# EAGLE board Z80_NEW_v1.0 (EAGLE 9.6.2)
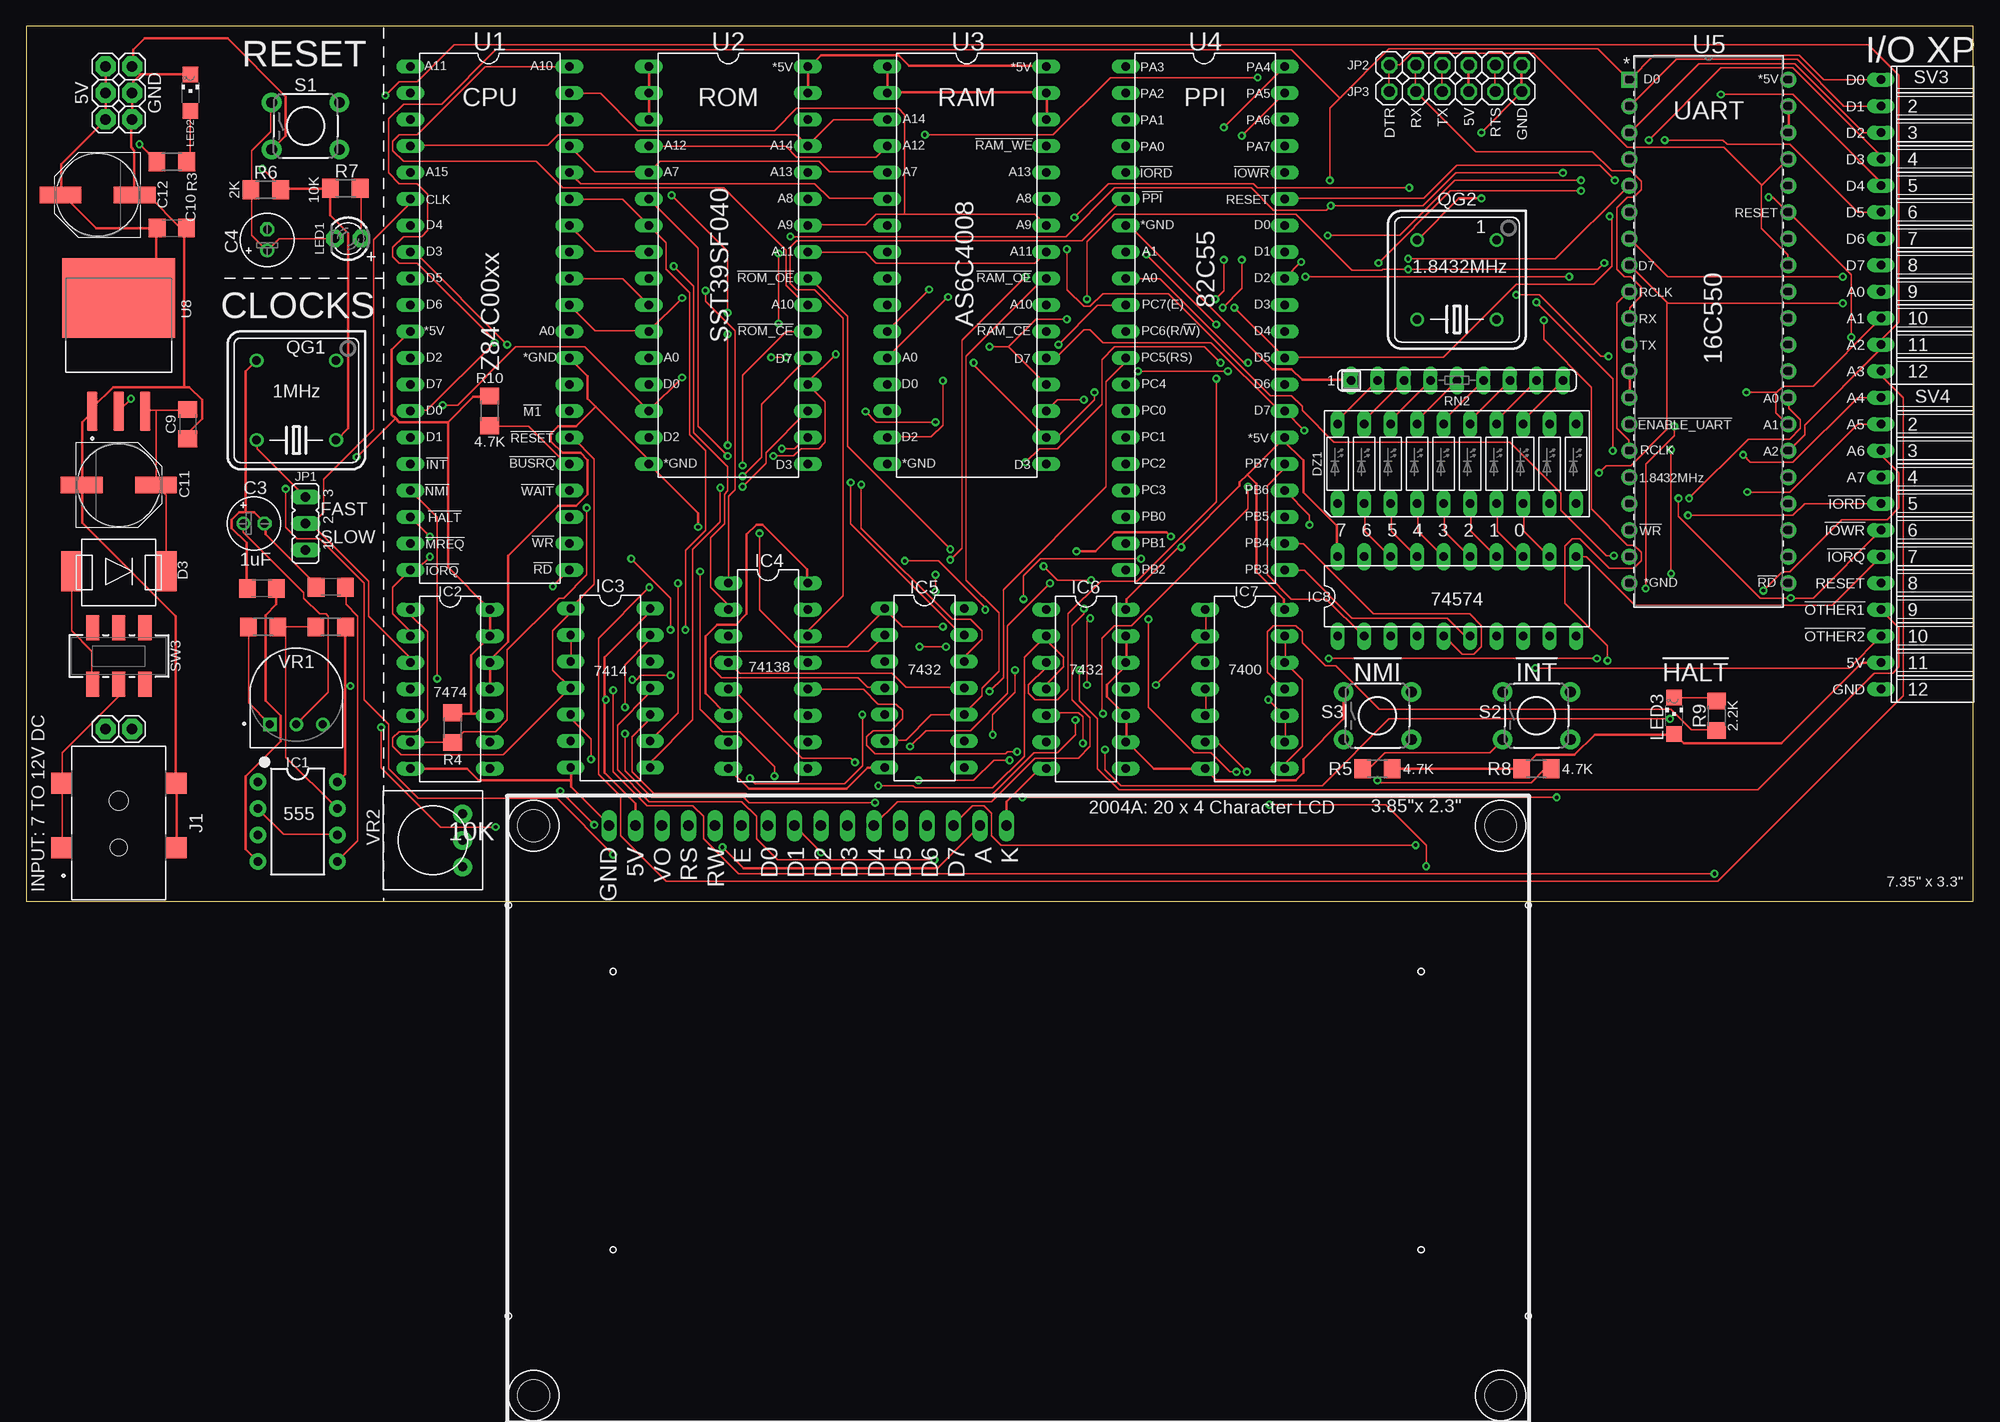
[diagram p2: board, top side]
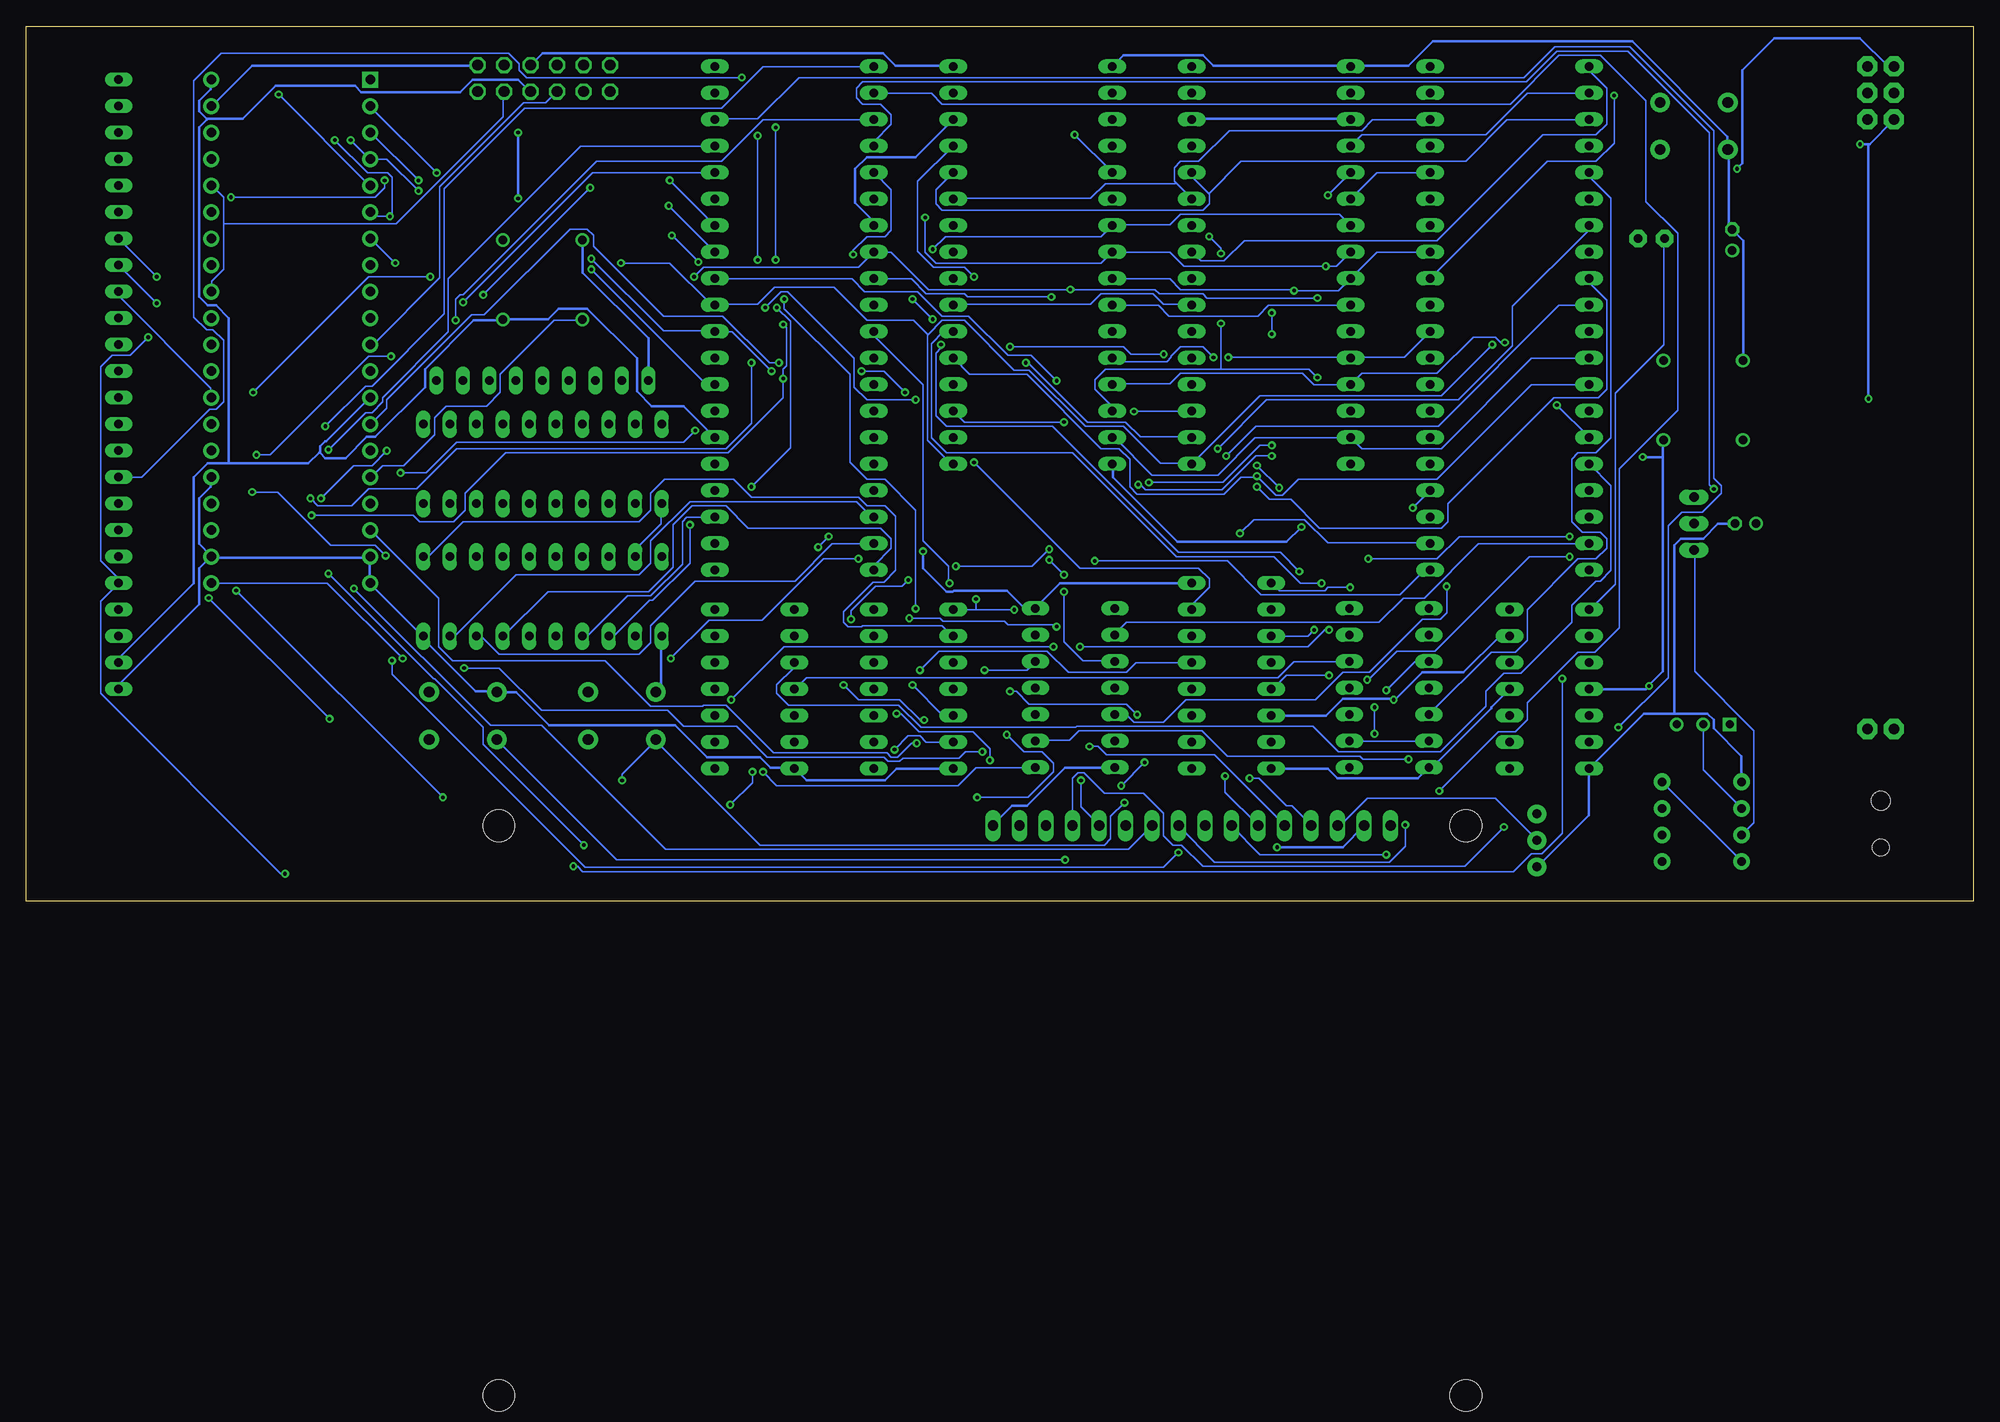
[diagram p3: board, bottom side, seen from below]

Size 186.67 x 83.87 mm. Coordinates in mm from the lower left corner, seen from the top.
Outline: 0,0 186.67,0 186.67,83.87 0,83.87 0,0
Copper layers (1*16): Top 0.035mm / dielectric 0.15mm / Bottom 0.035mm
Design rules "default": minimum track width 6mil, minimum drill 0.35mm, track to track 6mil, track to pad 6mil, pad to pad 6mil, via to via 6mil, smd to smd 6mil, copper to edge 40mil, drill to drill 6mil, minimum pad ring 10mil, minimum via ring 8mil, stop-mask expansion 4mil, vias tented up to drill 0mil, thermal gap 10mil
Net classes: 0 default: clearance 0.254 mm; 3 Power: width 0.254 mm, clearance 0.254 mm
tRestrict: area 17.8,0 to 19,81.3; area 11.4,81.3 to 19.1,82.5; area 0,81.3 to 6.3,82.5
bRestrict: area 17.8,0 to 19,81.3; area 11.4,81.3 to 19.1,82.5; area 0,81.3 to 6.3,82.5

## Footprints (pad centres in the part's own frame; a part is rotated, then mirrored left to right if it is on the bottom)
C1206 = smd 1.6 x 1.8: 1 -1.4,0; 2 1.4,0
E2-5 = drill 0.813 pad 1.27: + -1.016,0 | drill 0.813 pad 1.27 octagon: - 1.016,0
PANASONIC_F = smd 4 x 1.6: + 3.55,0; - -3.55,0
DIODE_5V5A = smd 1.93 x 3.81: A -4.572,0; C 4.572,0
LB10 = drill 0.813 long: 1 -11.43,-3.81; 2 -8.89,-3.81; 3 -6.35,-3.81; 4 -3.81,-3.81; 5 -1.27,-3.81; 6 1.27,-3.81; 7 3.81,-3.81; 8 6.35,-3.81; 9 8.89,-3.81; 10 11.43,-3.81; 11 11.43,3.81; 12 8.89,3.81; 13 6.35,3.81; 14 3.81,3.81; 15 1.27,3.81; 16 -1.27,3.81; 17 -3.81,3.81; 18 -6.35,3.81; 19 -8.89,3.81; 20 -11.43,3.81
DIP08 = drill 0.813 pad 1.626: 1 -3.81,-3.81; 2 -1.27,-3.81; 3 1.27,-3.81; 4 3.81,-3.81; 5 3.81,3.81; 6 1.27,3.81; 7 -1.27,3.81; 8 -3.81,3.81
DIL14 = drill 0.813 long: 1 -7.62,-3.81; 2 -5.08,-3.81; 3 -2.54,-3.81; 4 0,-3.81; 5 2.54,-3.81; 6 5.08,-3.81; 7 7.62,-3.81; 8 7.62,3.81; 9 5.08,3.81; 10 2.54,3.81; 11 0,3.81; 12 -2.54,3.81; 13 -5.08,3.81; 14 -7.62,3.81
DIL16 = drill 0.813 long: 1 -8.89,-3.81; 2 -6.35,-3.81; 3 -3.81,-3.81; 4 -1.27,-3.81; 5 1.27,-3.81; 6 3.81,-3.81; 7 6.35,-3.81; 8 8.89,-3.81; 9 8.89,3.81; 10 6.35,3.81; 11 3.81,3.81; 12 1.27,3.81; 13 -1.27,3.81; 14 -3.81,3.81; 15 -6.35,3.81; 16 -8.89,3.81
DIL20 = drill 0.813 long: 1 -11.43,-3.81; 2 -8.89,-3.81; 3 -6.35,-3.81; 4 -3.81,-3.81; 5 -1.27,-3.81; 6 1.27,-3.81; 7 3.81,-3.81; 8 6.35,-3.81; 9 8.89,-3.81; 10 11.43,-3.81; 11 11.43,3.81; 12 8.89,3.81; 13 6.35,3.81; 14 3.81,3.81; 15 1.27,3.81; 16 -1.27,3.81; 17 -3.81,3.81; 18 -6.35,3.81; 19 -8.89,3.81; 20 -11.43,3.81
SPARKFUN_PRT-12748 = smd 2 x 2: 1_1 -2.35,5.5; 1_2 3.8,5.5; 2 -2.35,-5.5; 3 3.8,-5.5 | hole 1.6: -2.35,0 | hole 1.8: 2.15,0
JP2 = drill 0.914 long: 1 -2.54,0; 2 0,0; 3 2.54,0
1X06 = drill 1.016 octagon: 1 -6.35,0; 2 -3.81,0; 3 -1.27,0; 4 1.27,0; 5 3.81,0; 6 6.35,0
1X01 = drill 1.016 pad 1.93 octagon: 1 0,0
LED3MM = drill 0.813 pad 1.676 octagon: A -1.27,0; K 1.27,0
CHIPLED_1206 = smd 1.5 x 1.5: A 0,-1.75; C 0,1.75
DIL08S = drill 0.813: 1 -3.81,-3.81; 4 3.81,-3.81; 5 3.81,3.81; 8 -3.81,3.81
R1206 = smd 1.6 x 1.803: 1 -1.422,0; 2 1.422,0
SIL9 = drill 0.813 long: 1 -10.16,0; 2 -7.62,0; 3 -5.08,0; 4 -2.54,0; 5 0,0; 6 2.54,0; 7 5.08,0; 8 7.62,0; 9 10.16,0
MOMENTARY_SWITCH = drill 1.016 pad 1.88: 1 -3.251,2.261; 2 3.251,2.261; 3 -3.251,-2.261; 4 3.251,-2.261
FE12W = drill 0.813 long: 1 -13.97,0; 2 -11.43,0; 3 -8.89,0; 4 -6.35,0; 5 -3.81,0; 6 -1.27,0; 7 1.27,0; 8 3.81,0; 9 6.35,0; 10 8.89,0; 11 11.43,0; 12 13.97,0
JS202011SCQN = smd 1.27 x 2.4: 1 -2.5,-2.7; 2 0,-2.7; 3 2.5,-2.7; 4 -2.5,2.7; 5 0,2.7; 6 2.5,2.7
DIL40 = drill 0.813 long: 1 -24.13,-7.62; 2 -21.59,-7.62; 3 -19.05,-7.62; 4 -16.51,-7.62; 5 -13.97,-7.62; 6 -11.43,-7.62; 7 -8.89,-7.62; 8 -6.35,-7.62; 9 -3.81,-7.62; 10 -1.27,-7.62; 11 1.27,-7.62; 12 3.81,-7.62; 13 6.35,-7.62; 14 8.89,-7.62; 15 11.43,-7.62; 16 13.97,-7.62; 17 16.51,-7.62; 18 19.05,-7.62; 19 21.59,-7.62; 20 24.13,-7.62; 21 24.13,7.62; 22 21.59,7.62; 23 19.05,7.62; 24 16.51,7.62; 25 13.97,7.62; 26 11.43,7.62; 27 8.89,7.62; 28 6.35,7.62; 29 3.81,7.62; 30 1.27,7.62; 31 -1.27,7.62; 32 -3.81,7.62; 33 -6.35,7.62; 34 -8.89,7.62; 35 -11.43,7.62; 36 -13.97,7.62; 37 -16.51,7.62; 38 -19.05,7.62; 39 -21.59,7.62; 40 -24.13,7.62
DIL32 = drill 0.813 long: 1 -19.05,-7.62; 2 -16.51,-7.62; 3 -13.97,-7.62; 4 -11.43,-7.62; 5 -8.89,-7.62; 6 -6.35,-7.62; 7 -3.81,-7.62; 8 -1.27,-7.62; 9 1.27,-7.62; 10 3.81,-7.62; 11 6.35,-7.62; 12 8.89,-7.62; 13 11.43,-7.62; 14 13.97,-7.62; 15 16.51,-7.62; 16 19.05,-7.62; 17 19.05,7.62; 18 16.51,7.62; 19 13.97,7.62; 20 11.43,7.62; 21 8.89,7.62; 22 6.35,7.62; 23 3.81,7.62; 24 1.27,7.62; 25 -1.27,7.62; 26 -3.81,7.62; 27 -6.35,7.62; 28 -8.89,7.62; 29 -11.43,7.62; 30 -13.97,7.62; 31 -16.51,7.62; 32 -19.05,7.62
N40A = drill 0.914 pad 1.524 square: 1 -15.24,48.26 | drill 0.914 pad 1.524: 2 -15.24,45.72; 3 -15.24,43.18; 4 -15.24,40.64; 5 -15.24,38.1; 6 -15.24,35.56; 7 -15.24,33.02; 8 -15.24,30.48; 9 -15.24,27.94; 10 -15.24,25.4; 11 -15.24,22.86; 12 -15.24,20.32; 13 -15.24,17.78; 14 -15.24,15.24; 15 -15.24,12.7; 16 -15.24,10.16; 17 -15.24,7.62; 18 -15.24,5.08; 19 -15.24,2.54; 20 -15.24,0; 21 0,0; 22 0,2.54; 23 0,5.08; 24 0,7.62; 25 0,10.16; 26 0,12.7; 27 0,15.24; 28 0,17.78; 29 0,20.32; 30 0,22.86; 31 0,25.4; 32 0,27.94; 33 0,30.48; 34 0,33.02; 35 0,35.56; 36 0,38.1; 37 0,40.64; 38 0,43.18; 39 0,45.72; 40 0,48.26
20X4LCD_2004A = drill 1 long: 1 -41.021,27.94; 2 -38.481,27.94; 3 -35.941,27.94; 4 -33.401,27.94; 5 -30.861,27.94; 6 -28.321,27.94; 7 -25.781,27.94; 8 -23.241,27.94; 9 -20.701,27.94; 10 -18.161,27.94; 11 -15.621,27.94; 12 -13.081,27.94; 13 -10.541,27.94; 14 -8.001,27.94; 15 -5.461,27.94; 16 -2.921,27.94 | hole 3.048: -48.26,-26.67; 44.45,-26.67; 44.45,27.94; -48.26,27.94
TO254P1524X483-4N = smd 3.79 x 0.99: 1 -6.4,2.54; 2 -6.4,0; 3 -6.4,-2.54 | smd 7.62 x 10.84: 4 4.48,0
TRIM_3352T-1-105LF = drill 0.76 pad 1.16 square: 1 -2.54,-2.87 | drill 0.76 pad 1.16: 2 0,-2.87; 3 2.54,-2.87
TRIM-3386 = drill 0.9 pad 1.778: 1 -2.54,-2.857; 2 0,-2.857; 3 2.54,-2.857

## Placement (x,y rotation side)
C1  0.01uF  [C1206]  29.21,30.1 180 top
C2  0.01uF  [C1206]  22.61,29.97 180 top
C3  1uF  [E2-5]  21.84,36.2 0 top
C4  10uF  [E2-5]  23.11,63.37 90 top
C9  100nF  [C1206]  15.49,45.72 270 top
C10  100nF  [C1206]  13.97,64.52 0 top
C11  100uF  [PANASONIC_F]  8.89,39.88 0 top
C12  100uF  [PANASONIC_F]  6.86,67.69 180 top
D3  D1  [DIODE_5V5A]  8.89,31.62 0 top
DZ1  [LB10]  137.16,41.91 0 top
IC1  555  [DIP08]  26.04,7.62 270 top
IC2  74HCT74N  [DIL14]  40.64,20.32 270 top
IC3  74HCT14N  [DIL14]  56.01,20.45 270 top
IC4  74HC138N  [DIL16]  71.12,21.59 270 top
IC5  74S32N  [DIL14]  86.11,20.45 270 top
IC6  7432N  [DIL14]  101.6,20.32 270 top
IC7  74HCT00N  [DIL14]  116.84,20.32 270 top
IC8  74HC574N  [DIL20]  137.16,29.21 0 top
J1  PRT-12748  [SPARKFUN_PRT-12748]  8.89,7.49 90 top
JP1  [JP2]  26.8,36.2 90 top
JP2  [1X06]  137.03,80.14 0 top
JP3  [1X06]  137.03,77.6 0 top
JP17  [1X01]  7.62,77.47 90 top
JP18  [1X01]  10.16,77.47 90 top
JP19  [1X01]  7.62,74.93 90 top
JP20  JP4  [1X01]  7.62,16.51 90 top
JP21  [1X01]  7.62,80.01 90 top
JP22  [1X01]  10.16,80.01 90 top
JP23  [1X01]  10.16,74.93 90 top
JP24  [1X01]  10.16,16.51 90 top
LED1  !RESET!  [LED3MM]  30.86,63.5 180 top
LED2  5v  [CHIPLED_1206]  15.75,77.47 0 top
LED3  !HALT!  [CHIPLED_1206]  157.99,17.78 0 top
QG1  [DIL08S]  25.91,48.01 180 top
QG2  1.8432MHz  [DIL08S]  137.16,59.56 180 top
R1  1k  [R1206]  29.21,26.29 0 top
R2  1k  [R1206]  22.73,26.29 0 top
R3  2K  [R1206]  13.97,70.87 180 top
R4  4.7k  [R1206]  40.89,16.64 90 top
R5  4.7k  [R1206]  129.54,12.7 0 top
R6  10k  [R1206]  22.99,68.2 0 top
R7  2.2k  [R1206]  30.61,68.33 180 top
R8  4.7k  [R1206]  144.78,12.7 0 top
R9  2K  [R1206]  162.05,17.78 270 top
R10  4.7k  [R1206]  44.45,46.99 270 top
RN2  330  [SIL9]  137.16,49.91 0 top
S1  MOMENTARY_SWITCH"  [MOMENTARY_SWITCH]  26.8,74.3 0 top
S2  MOMENTARY_SWITCH"  [MOMENTARY_SWITCH]  144.78,17.78 0 top
S3  MOMENTARY_SWITCH"  [MOMENTARY_SWITCH]  129.54,17.78 0 top
SV3  [FE12W]  177.8,64.77 270 top
SV4  [FE12W]  177.8,34.29 270 top
SW3  JS202011SCQN  [JS202011SCQN]  8.89,23.5 0 top
U1  [DIL40]  44.45,55.88 270 top
U2  SST39SF040_DIP32  [DIL32]  67.31,60.96 270 top
U3  ALLIANCE_AS6C4008  [DIL32]  90.17,60.96 270 top
U4  8255A  [DIL40]  113.03,55.88 270 top
U5  PC16550DN/NOPB  [N40A]  168.91,30.48 0 top
U6  20X4LCD_2004A  [20X4LCD_2004A]  96.9,-20.7 0 top
U8  LM1084ISX-5.0/NOPB  [TO254P1524X483-4N]  8.89,53.34 90 top
VR1  1000k  [TRIM_3352T-1-105LF]  25.91,19.81 0 top
VR2  10k  [TRIM-3386]  38.99,5.84 90 top

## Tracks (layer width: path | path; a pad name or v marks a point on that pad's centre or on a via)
1-100HZ
  Bottom 0.152: JP1.1 26.72,33.63 26.72,22.05 21.03,16.36 21.03,7.52 22.15,6.4 IC1.3
1.8432MHZ
  Bottom 0.152: QG2.5 133.4,55.68 136.04,55.68 141.22,50.49 141.22,48.77 142.54,47.45 146.41,47.45 147.52,46.33 147.52,44.7 150.47,41.76 152.5,41.76 153.62,40.64 U5.16
1MHZ
  Top 0.152: JP1.3 22.15,43.38 22.15,44.2 QG1.5
5V  (via drill 0.35)
  Top 0.254: 55.47,19.3 55.47,12.29 58.42,9.35 U6.2 | 55.47,19.3 55.47,23.37 59.74,27.64 59.74,28.04 IC3.14 | v66.75,5.18 68.78,3.15 87.38,3.15 91.44,7.21 U6.15 | 40.44,45.92 42.88,48.36 44.4,48.36 R10.1 | 40.44,45.92 35.76,45.92 35.41,46.28 | 35.41,46.28 35.05,46.63 35.05,52.83 U1.11 | 42.67,17.98 44.2,17.98 44.4,17.78 IC2.10 | 42.67,17.98 40.95,17.98 R4.2 | 42.67,17.98 42.67,23.57 44.4,25.3 IC2.13 44.5,25.4 44.5,27.94 IC2.14 44.4,28.04 40.44,32 40.44,45.92 | IC4.16 74.88,30.48 74.88,31.8 70.61,36.07 70,36.07 69.09,35.15 69.09,27.53 68.07,26.52 66.24,26.52 65.13,25.4 65.13,19.91 67.26,17.78 IC4.6 | v55.58,19.3 55.47,19.3 | U8.4 8.94,57.91 12.5,61.47 12.5,64.52 C10.1 6.71,64.52 3.45,67.77 C12.+ 3.35,67.77 3.35,70.61 7.62,74.88 JP19.1 JP17.1 JP21.1 | v10.87,72.54 12.5,70.92 R3.2 | v10.06,48.16 8.94,47.04 U8.2 | C2.1 23.98,29.97 23.98,28.45 22.96,27.43 22.96,19.2 24.38,17.78 24.38,15.34 21.03,11.99 21.03,4.98 22.15,3.86 IC1.4 | 30.58,20.62 30.58,12.19 29.87,11.48 IC1.8 | 30.58,20.62 30.58,26.21 R1.2 | 30.58,20.62 v31.09,20.62 | QG1.8 29.77,44.2 30.89,45.31 30.89,64.01 29.16,65.73 29.16,68.17 R7.2 29.16,68.28 24.49,68.28 R6.2 24.49,68.38 v22.66,70.21 | v31.7,42.57 35.41,46.28 | U2.31 74.98,77.52 74.98,79.96 U2.32 75.08,79.96 76.2,81.08 83.62,81.08 84.63,80.06 97.74,80.06 U3.32 | JP3.4 138.28,77.62 138.28,80.06 JP2.4 | R5.2 R8.1 143.46,12.7 144.78,14.02 148.44,14.02 150.37,15.95 157.99,15.95 LED3.A 158.09,15.95 158.9,15.14 168.25,15.14 175.97,22.86 SV4.11 | U5.13 153.72,48.26 153.72,50.8 U5.12 | 110.59,34.09 116.33,39.83 116.33,40.13 117.09,40.89 | 110.59,34.09 105.46,28.96 105.46,27.94 IC6.14
  Top 0.254: 117.09,40.89 U4.26 120.5,44.2 122.43,42.27 122.43,39.22 125.68,35.97 125.68,33.02 IC8.20 | 117.09,40.89 117.96,40.03 117.96,31.6 120.6,28.96 120.6,27.94 IC7.14 | v100.69,33.53 102.51,33.53 104.34,35.36 109.32,35.36 v109.73,34.95 | 110.59,34.09 v110.74,33.93
  Bottom 0.254: v66.75,5.18 60.45,5.18 58.42,7.21 U6.2 | IC4.16 87.58,30.48 89.92,28.14 IC5.14 90.02,28.14 91.03,28.14 92.66,29.77 97.74,29.77 97.84,29.67 98.45,29.67 100.69,31.9 v100.69,33.53 | IC4.6 62.08,17.78 60.45,19.41 55.58,19.41 | 55.58,19.41 55.37,19.41 52.83,21.95 48.87,21.95 45.41,25.4 IC2.13 | v55.58,19.3 55.58,19.41 | 10.06,72.54 9.96,72.54 7.62,74.88 JP19.1 | 10.06,72.54 v10.87,72.54 | 10.06,72.54 v10.06,48.16 | IC2.4 31.39,20.32 v31.09,20.62 31.09,20.73 29.77,22.05 29.77,42.57 | 29.77,42.57 29.77,44.2 QG1.8 | IC1.4 22.25,3.86 29.77,11.38 IC1.8 | v22.66,70.21 22.15,70.71 22.15,79.65 19.1,82.7 10.87,82.7 8.23,80.06 7.62,80.06 JP21.1 | 29.77,42.57 v31.7,42.57 | 169.37,74.98 170.08,75.69 170.08,76.71 168.96,77.83 168.96,78.74 U5.40 | 169.37,74.98 165.91,74.98 162.76,78.13 155.14,78.13 154.53,77.52 145.09,77.52 143.87,78.74 139.5,78.74 138.38,77.62 JP3.4 | JP2.4 137.16,81.28 104.55,81.28 103.33,80.06 97.84,80.06 U3.32 | U4.26 123.65,47.45 126.69,47.45 128.12,48.87 128.12,52.02 132.89,56.79 135.64,56.79 136.65,55.78 140.92,55.78 QG2.8 141.02,55.68 143.76,55.68 148.44,51 148.44,49.28 153.21,44.5 154.03,44.5 156.06,42.47 157.99,42.47 158.5,42.98 | 158.5,42.98 158.5,43.59 157.99,44.09 157.89,44.09 153.72,48.26 U5.13 | SV4.11 177.8,23.27 170.59,30.48 170.59,40.64 169.27,41.96 167.23,41.96 | 167.23,41.96 159.61,41.96 158.6,42.98 158.5,42.98 | 167.23,41.96 167.23,55.88 168.45,57.1 169.27,57.1 170.08,57.91 170.08,74.17 169.37,74.88 169.37,74.98 | v110.74,33.93 v109.73,34.95
12V-0.7V
  Top 0.152: 12.5,47.04 11.48,47.04 U8.3 | 12.5,47.04 15.44,47.04 C9.1 | D3.C 13.41,31.7 13.41,38.91 12.5,39.83 C11.+ 12.5,39.93 12.5,47.04
!BUSRQ!
  Top 0.152: R10.2 44.5,45.52 48.16,45.52 51.71,41.96 52.02,41.96 U1.25
!CTS-RTS!
  Top 0.152: JP3.5 140.82,77.62 140.82,80.06 JP2.5
  Bottom 0.152: 167.74,64.92 167.74,67.46 168.86,68.58 U5.36 | 167.74,64.92 167.74,60.55 168.86,59.44 168.86,58.42 U5.32 | 167.74,64.92 151.18,64.92 140.92,75.18 140.92,77.52 JP3.5
!DSR-DTR!
  Top 0.152: JP3.1 130.66,77.62 130.66,80.06 JP2.1 130.76,80.16 131.67,80.16 132.79,81.28 144.47,81.28 153.52,72.24 162.76,72.24 166.37,68.63 | 166.37,68.63 168.86,71.12 U5.37 | 166.37,68.63 166.32,68.58 166.32,64.52 168.86,61.98 168.86,60.96 U5.33
!ENABLE_IO!
  Top 0.152: IC5.11 89.92,20.52 84.33,20.52 83.01,21.84 68.38,21.84 67.36,22.86 IC4.4
!ENABLE_PPI!
  Top 0.152: IC4.14 74.98,25.4 74.98,25.91 78.33,29.26 78.33,55.88 75.59,58.62 73.86,58.62 73.25,59.23 73.25,62.69 73.86,63.3 101.19,63.3 105.16,67.26 105.36,67.26 U4.6
!ENABLE_UART!  (via drill 0.35)
  Top 0.152: v95.81,42.06 97.13,43.38 98.86,43.38 103.12,47.65 103.12,51.92 104.34,53.14 112.98,53.14 v114.5,51.61
  Bottom 0.152: v95.81,42.06 85.65,31.9 74.27,31.9 73.25,30.89 73.25,30.07 74.88,28.45 74.88,27.94 IC4.15 | v114.5,51.61 115.42,51.61 119.89,56.08 125.58,56.08 132.28,62.79 132.28,63.8 132.89,64.41 134.52,64.41 142.75,56.19 143.97,56.19 152.09,48.06 152.09,47.24 153.62,45.72 U5.14
!HALT!  (via drill 0.35)
  Top 0.152: v38.71,34.95 U1.18 | v58.01,32.82 61.77,29.06 v61.77,26.01 | v88.19,24.38 v85.65,24.38 | v119.08,19.3 120.6,17.78 IC7.10 120.7,17.78 120.7,15.24 IC7.9
  Bottom 0.152: v38.71,34.95 49.28,34.95 51.41,32.82 v58.01,32.82 | v61.77,26.01 62.18,26.01 63.8,24.38 v85.65,24.38 | v88.19,24.38 114,24.38 v119.08,19.3
!INT!
  Bottom 0.152: U1.16 34.75,39.83 34.75,31.7 35.76,30.68 36.17,30.68 38.51,28.35 38.51,26.72 43.38,21.84 45.01,21.84 46.74,20.12 46.74,18.69 51.1,14.33 60.86,14.33 63.3,16.76 85.95,16.76 86.06,16.66 100.89,16.66 103.02,18.8 113.59,18.8 114.71,19.91 114.71,20.73 113.08,22.35 113.08,22.86 IC7.3
!IORD!  (via drill 0.35)
  Top 0.152: v114.1,50.09 114.1,38.3 106.48,30.68 103.02,30.68 99.87,27.53 99.87,20.32 98.86,19.3 96.72,19.3 96.11,19.91 96.11,20.73 97.74,22.35 97.74,22.86 IC6.3 | v107.39,61.98 v114.1,55.27 | SV4.5 170.49,38.1 169.37,36.98 v159.31,36.98
  Bottom 0.152: v114.1,55.27 113.79,54.97 113.79,51.31 114.1,51 v114.1,50.09 114.1,48.26 119.38,42.98 140.72,42.98 144.58,39.12 144.58,37.49 145.69,36.37 148.95,36.37 149.56,36.98 v159.31,36.98 | v107.39,61.98 107.39,62.38 106.07,63.7 104.34,63.7 103.73,64.31 103.73,68.17 U4.5
!IORQ!  (via drill 0.35)
  Top 0.152: IC8.11 149.56,33.02 154.23,28.35 173.13,28.35 SV4.7 | IC2.2 36.78,25.4 36.78,25.91 35.15,27.53 35.15,30.07 U1.20 36.88,31.8 37.49,31.8 v38.71,33.02 | IC4.5 67.77,20.32 74.37,13.72 79.05,13.72 v79.45,13.31 | v81.69,11.07 85.04,11.07 85.24,10.87 92.66,10.87 95.71,13.92 95.71,23.37 97.74,25.4 IC6.2 97.64,25.2 99.47,23.37 99.47,22.45 97.84,20.83 97.84,20.32 IC6.4 | v58.12,21.23 58.52,21.23 58.93,21.64 v61.77,21.64
  Bottom 0.152: v81.69,11.07 v79.45,13.31 | v38.71,33.02 42.57,33.02 51.61,23.98 55.27,23.98 58.01,21.23 v58.12,21.23 | v61.77,21.64 65.84,21.64 67.16,20.32 IC4.5 | IC8.11 148.13,33.02 144.78,36.37 127.91,36.37 126.8,37.49 126.8,39.12 125.48,40.44 118.87,40.44 117.14,38.71 106.88,38.71 106.07,37.9 104.34,37.9 103.33,36.88 103.33,31.7 104.44,30.58 105.46,30.58 108.31,27.74 108.31,26.72 107.9,26.31 106.58,26.31 106.48,26.42 98.86,26.42 97.84,25.4 IC6.2
!IOWR!  (via drill 0.35)
  Top 0.152: v103.43,14.53 103.43,12.6 104.95,11.07 124.26,11.07 130.66,17.48 v157.58,17.48 | SV4.6 171.3,29.06 v169.16,29.06 166.22,29.06 158.39,36.88 v158.39,38.61 | v144.78,57.4 152.09,50.09 v152.09,43.18
  Bottom 0.152: IC6.6 100.38,15.24 100.99,15.85 102.11,15.85 v103.43,14.53 | v169.16,29.06 v157.58,17.48 | v144.78,57.4 132.38,69.8 120.7,69.8 U4.36 | v152.09,43.18 153.52,41.76 155.25,41.76 v158.39,38.61
!MREQ!
  Top 0.152: IC5.4 82.3,20.52 80.67,20.52 79.76,21.44 66.65,21.44 65.63,22.45 65.63,23.27 66.34,23.98 80.77,23.98 82.3,25.5 IC5.2
  Bottom 0.152: U1.19 36.88,34.24 47.45,34.24 52.63,29.06 54.66,29.06 57,26.72 81.18,26.72 82.3,25.6 IC5.2
!NMI!  (via drill 0.35)
  Top 0.152: IC7.6 114.2,15.24 v117.04,12.39 | v119.18,9.25 130.35,9.25 134.21,5.38 v134.21,3.35 | v39.42,21.34 39.42,36.78 U1.17
  Bottom 0.152: v117.04,12.39 117.04,11.38 v119.18,9.25 | v134.21,3.35 133.81,3.35 133.3,2.85 44.09,2.85 42.37,4.57 41.35,4.57 39.42,6.5 v39.42,21.34
!OTHER1!  (via drill 0.35)
  Top 0.152: v100.99,22.15 100.99,19.2 102.72,17.48 102.72,12.7 104.75,10.67 166.01,10.67 177.19,21.84 178.92,21.84 179.53,22.45 179.53,26.21 SV4.9
  Bottom 0.152: IC4.13 80.26,22.86 81.18,21.95 86.77,21.95 88.8,23.98 99.16,23.98 v100.99,22.15
!OTHER2!  (via drill 0.35)
  Top 0.152: IC4.12 80.26,20.32 81.69,18.9 83.41,18.9 84.02,18.29 84.02,17.48 82.91,16.36 81.18,16.36 80.57,15.75 80.57,14.94 81.38,14.12 93.88,14.12 94.08,14.33 v95,14.33 | v144.68,22.35 174.75,22.35 SV4.10
  Bottom 0.152: v95,14.33 96.62,14.33 97.23,13.72 102.62,13.72 102.92,13.41 104.04,13.41 104.44,13.82 115.62,13.82 118.57,16.76 123.65,16.76 125.17,18.29 137.26,18.29 141.33,22.35 v144.68,22.35
!RAM_CE!  (via drill 0.35)
  Top 0.152: v62.48,30.48 62.48,18.09 59.84,15.44 IC3.9
  Bottom 0.152: IC3.6 52.22,15.34 59.74,15.34 IC3.9 | v62.48,30.48 64.52,30.48 67.06,33.02 76.4,33.02 86.36,42.98 98.45,42.98 99.87,44.4 99.87,53.44 98.75,54.56 97.84,54.56 U3.22
!RAM_WE!  (via drill 0.35)
  Top 0.152: v87.17,31.29 v87.17,29.67 | v88.59,32.72 89.71,33.83 89.71,53.75 v95.81,59.84
  Bottom 0.152: v87.17,29.67 87.17,24.89 85.34,23.06 82.3,23.06 IC5.3 | v88.59,32.72 v87.17,31.29 | v95.81,59.84 96.72,60.76 99.67,60.76 101.19,62.28 101.19,68.99 U3.29
!RD!  (via drill 0.35)
  Top 0.152: U1.21 v50.49,30.18 | v91.95,27.94 91.95,28.14 87.48,32.61 v84.23,32.61 | v124.87,23.27 v150.57,23.27 | v106.88,32.82 97.23,32.82 95.61,31.19 v95.61,28.96
  Bottom 0.152: v50.49,30.18 50.49,27.64 51.1,27.03 52.83,27.03 57.91,21.95 60.45,21.95 63.09,19.3 75.49,19.3 77.62,17.17 80.47,17.17 81.18,17.88 82.3,17.88 IC5.5 | v91.95,27.94 95.61,27.94 | 95.61,27.94 IC6.1 | v84.23,32.61 71.53,32.61 68.28,29.36 54.97,29.36 52.63,31.7 52.12,31.7 U1.21 | U5.21 157.78,30.48 v150.57,23.27 | v124.87,23.27 121.21,26.92 116.13,26.92 110.24,32.82 v106.88,32.82 | 95.61,27.94 v95.61,28.96
!RESET!
  Top 0.152: LED1.K 24.28,63.5 23.16,62.38 C4.+ 23.06,62.38 21.64,63.8 21.64,68.17 R6.1 21.64,68.28 21.64,71.93 23.47,73.76 23.47,76.5 S1.1 | IC2.1 36.88,27.94 36.88,27.43 38.51,25.81 38.51,17.37 37.39,16.26 35.76,16.26 35.15,15.65 35.15,14.83 35.97,14.02 45.72,14.02 52.12,20.42 IC3.4 50.49,22.15 50.49,25.91 52.12,27.53 52.12,28.04 IC3.1 52.22,28.14 54.46,30.38 54.46,42.37 52.43,44.4 52.12,44.4 U1.26
  Bottom 0.152: LED1.K 29.67,63.5 29.67,53.34 34.34,48.67 34.34,30.38 36.78,27.94 IC2.1
!ROM-RAM_OE!
  Top 0.152: IC5.6 82.3,15.44 84.33,15.44 86.77,17.88 89.92,17.88 IC5.10 89.92,17.98 91.64,19.71 91.64,20.42 93.27,22.05 93.27,27.64 90.12,30.79 90.12,52.22 97.54,59.64 97.74,59.64 U3.24
!ROM_CE!  (via drill 0.35)
  Top 0.152: v66.55,39.62 66.55,36.37 63.91,33.73 63.91,17.37 59.84,13.31 59.84,12.9 IC3.8 | v68.68,41.76 68.68,50.39 72.85,54.56 74.88,54.56 U2.22
  Bottom 0.152: v68.68,41.76 v66.55,39.62
!ROM_OE!  (via drill 0.35)
  Top 0.152: v116.03,12.39 115.42,12.39 113.59,14.22 111.96,14.22 107.59,18.59 v107.59,27.03 | v102.11,30.79 98.86,30.79 v97.54,32.11 | v88.59,33.73 78.74,43.59 78.74,56.08 75.18,59.64 74.98,59.64 U2.24
  Bottom 0.152: v116.03,12.39 114.71,11.07 97.33,11.07 95.61,12.8 89.92,12.8 IC5.8 | v107.59,27.03 107.59,27.84 105.26,30.18 102.72,30.18 v102.11,30.79 | v97.54,32.11 90.22,32.11 v88.59,33.73
!WAIT!  (via drill 0.35)
  Top 0.152: IC2.6 40.84,15.24 R4.1 40.95,15.24 41.96,16.26 45.01,16.26 46.13,17.37 46.13,24.08 51.1,29.06 51.51,29.06 53.75,31.29 v53.75,37.69
  Bottom 0.152: v53.75,37.69 U1.24
!WR!  (via drill 0.35)
  Top 0.152: v101.7,20.73 101.7,26.82 v102.01,27.13 | v87.88,26.31 84.02,26.31 82.3,28.04 IC5.1 82.3,27.94 78.74,24.38 73.86,24.38 70.31,27.94 v70.31,35.26 | v101.3,15.14 101.3,17.68 100.89,18.09 98.15,18.09 97.84,17.78 IC6.5
  Bottom 0.152: IC6.5 98.75,17.78 v101.7,20.73 | v102.01,27.13 99.06,27.13 98.75,26.82 92.86,26.82 92.56,26.52 88.09,26.52 v87.88,26.31 | v70.31,35.26 68.99,36.58 64.11,36.58 61.87,34.34 52.12,34.34 U1.22 | v101.3,15.14 101.8,15.14 103.12,13.82 103.73,13.82 104.14,14.22 115.01,14.22 119.58,18.8 121.72,18.8 121.82,18.69 126.8,18.69 131.17,23.06 145.8,23.06 147.12,24.38 147.12,29.06 153.62,35.56 U5.18
A0  (via drill 0.35)
  Top 0.152: v88.39,57.91 U3.12 | v72.85,52.12 v71.42,52.12 | v159.41,38.61 165.1,44.3 169.06,44.3 170.08,45.31 170.08,46.13 168.96,47.24 168.96,48.26 U5.28 | v117.14,51.61 116.74,51.61 108.71,59.64 105.46,59.64 U4.9
  Bottom 0.152: SV3.9 177.8,58.01 168.96,49.17 168.96,48.26 U5.28 | U1.30 54.56,52.12 59.64,52.12 U2.12 59.74,52.12 v71.42,52.12 | v88.39,57.91 96.42,57.91 96.72,58.22 100.38,58.22 101.8,59.64 105.36,59.64 U4.9 | v72.85,52.12 73.86,53.14 76,53.14 76.91,52.22 76.91,52.12 77.32,51.71 82.19,51.71 U3.12 | v159.41,38.61 158.7,37.9 155.45,37.9 153.82,39.52 149.25,39.52 145.39,43.38 119.58,43.38 117.14,45.82 v117.14,51.61
A1  (via drill 0.35)
  Top 0.152: SV3.10 171.3,49.38 168.45,49.38 167.79,48.72 | 167.79,48.72 167.74,48.67 167.74,46.84 168.86,45.72 U5.27 | U1.31 54.56,54.66 59.64,54.66 U2.11 v62.89,57.81 | v86.56,58.62 U3.11 | v164.9,48.77 167.74,48.77 167.79,48.72 | v122.63,59.84 v147.93,59.84
  Bottom 0.152: v62.89,57.81 73.46,57.81 73.86,58.22 78.03,58.22 78.44,58.62 v86.56,58.62 100.18,58.62 103.73,62.18 105.36,62.18 U4.8 106.88,60.76 121.72,60.76 v122.63,59.84 | v164.9,48.77 153.82,59.84 v147.93,59.84
A2  (via drill 0.35)
  Top 0.152: U5.26 168.96,43.18 170.49,44.7 170.49,45.62 177.8,52.93 SV3.11 177.8,53.75 179.53,55.47 179.53,79.15 176.58,82.09 41.05,82.09 37.49,78.54 35.76,78.54 v34.44,77.22 | U2.10 57.2,59.64 52.12,59.64 U1.32
  Bottom 0.152: U3.10 82.5,57.1 78.13,57.1 77.11,56.08 68.58,56.08 67.56,57.1 59.74,57.1 U2.10 | v34.44,77.22 34.44,72.64 36.17,70.92 40.84,70.92 U1.32
A3  (via drill 0.35)
  Top 0.152: v65.13,58.52 65.13,57.51 67.97,54.66 67.97,39.42 67.36,38.81 67.36,30.48 IC4.1 | SV3.12 177.8,50.39 179.93,48.26 179.93,19.71 162.15,1.93 61.37,1.93 57,6.3 57,10.06 54.86,12.19 54.86,25.2 v59.74,30.07
  Bottom 0.152: U1.33 52.12,62.18 57.2,62.18 U2.9 60.86,58.52 v65.13,58.52 65.23,58.62 76,58.62 77.01,59.64 82.5,59.64 U3.9 | v59.74,30.07 61.87,30.07 62.18,29.77 66.55,29.77 67.26,30.48 IC4.1
A4  (via drill 0.35)
  Top 0.152: U1.34 54.56,62.28 59.64,62.28 U2.8 | v62.08,60.86 64.01,58.93 64.01,44.91 67.26,41.66 67.26,39.32 66.95,39.01 66.95,36.17 65.63,34.85 65.63,30.07 67.26,28.45 67.26,27.94 IC4.2 | SV4.1 175.56,48.26 169.37,42.06 165.3,42.06 v164.59,42.77 | v151.69,52.22 150.98,52.22 145.09,58.12 v142.85,58.12 | v132.59,68.38 118.06,68.38 117.65,68.78 103.73,68.78 v100.48,65.53
  Bottom 0.152: U2.8 61.06,60.86 v62.08,60.86 75.69,60.86 77.01,62.18 82.5,62.18 U3.8 83.62,61.16 99.47,61.16 100.48,62.18 v100.48,65.53 | v164.59,42.77 163.27,42.77 153.82,52.22 v151.69,52.22 | v132.59,68.38 v142.85,58.12
A5  (via drill 0.35)
  Top 0.152: v63.2,26.01 63.2,33.63 65.13,35.56 65.13,43.18 63.6,44.7 63.6,58.32 61.37,60.55 61.37,63.09 U2.7 57.2,67.26 52.12,67.26 U1.35 | SV4.2 175.56,45.72 169.06,39.22 v165,39.22 | v152.2,33.12 151.49,33.12 147.12,37.49 147.12,39.12 142.24,43.99 125.37,43.99 122.33,47.04 122.33,47.45 121.31,48.46 119.28,48.46 109.53,58.22 103.23,58.22 102.01,57 101.4,57 99.77,58.62 v99.77,62.48
  Bottom 0.152: IC4.3 63.8,25.4 v63.2,26.01 | U2.7 60.76,65.84 76,65.84 77.01,64.82 82.5,64.82 U3.7 83.62,63.7 98.55,63.7 v99.77,62.48 | v165,39.22 162.56,39.22 157.48,34.14 153.21,34.14 v152.2,33.12
A6  (via drill 0.35)
  Top 0.152: IC5.12 89.92,23.37 91.64,25.09 91.64,25.91 90.53,27.03 88.8,27.03 80.06,35.76 v80.06,39.93 | v67.26,42.67 64.41,45.52 64.41,62.59 U2.6 | SV4.3 177.8,42.77 179.53,41.05 179.53,37.69 178.41,36.58 174.04,36.58 169.06,31.6 168.35,31.6 v166.52,29.77 | v95.5,9.96 v146.71,9.96 | v92.66,15.95 92.66,17.88 94.79,20.02 v94.79,22.15 | U1.36 53.14,68.78 75.59,68.78 77.01,67.36 82.5,67.36 U3.6
  Bottom 0.152: v80.06,39.93 79.86,39.93 79.35,39.42 72.03,39.42 68.78,42.67 v67.26,42.67 | v146.71,9.96 v166.52,29.77 | v95.5,9.96 90.63,9.96 88.19,12.39 88.19,13.21 89.31,14.33 91.03,14.33 v92.66,15.95 | v94.79,22.15 90.73,22.15 89.92,22.96 IC5.12 | U2.6 57.2,69.8 52.12,69.8 U1.36
A7  (via drill 0.35)
  Top 0.152: U1.37 54.56,69.9 59.64,69.9 U2.5 60.76,70.92 76,70.92 77.01,69.9 82.5,69.9 U3.5 | v79.05,40.13 79.05,36.17 89.61,25.6 89.92,25.6 IC5.13 | v67.26,54.36 v67.26,43.69 | v67.26,56.39 67.26,62.28 v61.87,67.67 | v118.06,78.94 103.94,78.94 98.45,73.46 v86.16,73.46
  Bottom 0.152: v79.05,40.13 71.93,40.13 68.38,43.69 v67.26,43.69 | v67.26,56.39 v67.26,54.36 | U2.5 v61.87,67.67 | SV4.4 175.56,40.64 169.06,47.14 168.45,47.14 167.74,47.85 167.74,53.75 168.76,54.76 169.37,54.76 170.59,55.98 170.59,78.64 167.94,81.28 140.41,81.28 139.4,80.26 139.4,79.65 138.68,78.94 v118.06,78.94 | U3.5 v86.16,73.46
A8
  Bottom 0.152: U2.27 76.45,68.83 | 76.45,68.83 76.61,68.99 76.61,70.31 76,70.92 74.27,70.92 71.32,73.86 58.62,73.86 57.61,74.88 52.12,74.88 U1.38 | U3.27 97.74,67.36 84.63,67.36 83.21,68.78 76.5,68.78 76.45,68.83
A9
  Top 0.152: 84.23,65.84 96.72,65.84 U3.26 | 84.23,65.84 81.48,65.84 80.47,64.82 74.98,64.82 U2.26 | 84.23,65.84 84.23,75.39 83.62,76 73.86,76 71.73,73.86 58.62,73.86 55.07,77.42 52.12,77.42 U1.39
A10
  Top 0.152: U1.40 52.02,79.96 43.99,79.96 37.49,73.46 35.76,73.46 35.15,72.85 35.15,71.93 36.17,70.92 48.87,70.92 51.41,68.38 66.85,68.38 72.85,62.38 72.85,59.03 74.68,57.2 74.88,57.2 U2.23
  Bottom 0.152: U3.23 97.74,57.2 84.63,57.2 83.62,58.22 78.64,58.22 77.62,57.2 74.98,57.2 U2.23
A11
  Top 0.152: U3.25 96.72,61.16 81.48,61.16 80.47,62.18 74.98,62.18 U2.25
  Bottom 0.152: U2.25 74.07,61.37 71.83,61.37 69.9,63.3 51.41,63.3 41.25,73.46 36.17,73.46 35.15,74.47 35.15,77.93 36.78,79.55 36.78,79.96 U1.1
A12
  Top 0.152: U3.4 81.48,71.32 73.86,71.32 72.85,72.34 59.74,72.34 U2.4
  Bottom 0.152: U2.4 58.62,73.46 46.74,73.46 42.77,77.42 36.88,77.42 U1.2
A13
  Bottom 0.152: 73.3,67.82 73.25,67.77 73.25,66.85 73.86,66.24 98.86,66.24 99.47,66.85 99.47,68.17 U3.28 | 73.3,67.82 74.88,69.39 74.88,69.8 U2.28 | 73.3,67.82 70.21,70.92 48.67,70.92 44.7,74.88 36.88,74.88 U1.3
A14
  Top 0.152: U1.4 36.88,72.44 49.99,72.44 51,73.46 73.86,73.46 U2.29 77.42,74.88 82.5,74.88 U3.3
A15  (via drill 0.35)
  Top 0.152: v54.15,13.61 54.15,15.54 52.22,17.48 52.22,17.88 IC3.5
  Bottom 0.152: v54.15,13.61 58.52,13.61 58.83,13.92 71.53,13.92 73.97,16.36 85.75,16.36 86.67,15.44 89.92,15.44 IC5.9 | IC3.5 46.23,23.88 43.89,23.88 42.77,24.99 42.77,27.94 37.9,32.82 36.17,32.82 35.15,33.83 35.15,34.75 35.76,35.36 37.49,35.36 38.51,36.37 38.51,42.37 37.9,42.98 36.17,42.98 34.75,44.4 34.75,67.36 36.78,69.39 36.78,69.8 U1.5
ADJUST
  Bottom 0.152: U6.3 60.96,7.32 60.66,7.32 58.12,9.86 45.82,9.86 41.86,5.89 VR2.2
CLK
  Top 0.152: IC2.3 36.78,22.86 36.78,23.37 32.82,27.33 32.82,30.68 27.33,36.17 26.82,36.17 JP1.2 27.43,36.17 28.55,37.29 28.55,40.44 33.33,45.21 33.33,63.4 36.78,66.85 36.78,67.26 U1.6
D0  (via drill 0.35)
  Top 0.152: U1.14 36.88,47.04 38.41,47.04 v44.91,53.54 44.81,53.54 44.81,53.85 37.49,61.16 35.76,61.16 35.15,61.77 35.15,62.69 36.17,63.7 37.9,63.7 38.51,64.31 38.51,67.77 37.49,68.78 35.76,68.78 34.75,69.8 34.75,74.98 36.17,76.4 39.83,76.4 45.01,81.58 121.31,81.58 125.93,76.96 | v124.97,69.09 124.97,76 125.93,76.96 | 125.93,76.96 130.66,81.69 150.67,81.69 153.62,78.74 U5.1 153.72,78.74 156.06,81.08 169.98,81.08 172.31,78.74 SV3.1
  Bottom 0.152: v44.91,53.54 45.31,53.54 45.82,54.05 47.95,54.05 51.41,50.6 58.62,50.6 U2.13 59.74,49.48 63.2,49.48 64.31,50.6 76,50.6 77.01,49.58 82.5,49.58 U3.13 | v124.97,69.09 U4.34
D1  (via drill 0.35)
  Top 0.152: v39.93,47.55 41.35,47.55 46.94,53.14 53.54,53.14 U2.14 v62.89,50.19 | v147.32,69.8 137.06,69.8 133.91,66.65 v125.07,66.65 124.66,66.24 119.58,66.24 117.45,68.38 104.34,68.38 99.67,63.7 v73.25,63.7 | SV3.2 174.24,76.2 169.77,80.67 158.19,80.67 153.72,76.2 U5.2 | v72.14,62.08 v72.14,55.37
  Bottom 0.152: v39.93,47.55 U1.15 | 72.14,51 63.7,51 v62.89,50.19 | 72.14,51 83.21,51 84.23,49.99 84.23,49.07 82.6,47.45 82.6,47.04 U3.14 | v125.07,66.65 U4.33 | v147.32,69.8 153.72,76.2 U5.2 | v72.14,55.37 72.14,51 | v72.14,62.08 72.14,62.59 v73.25,63.7
D2  (via drill 0.35)
  Top 0.152: SV3.3 176.17,73.66 169.57,80.26 160.32,80.26 153.72,73.66 U5.3 | v87.88,49.89 87.88,45.62 86.77,44.5 82.6,44.5 U3.15 | v149.05,69.09 136.96,69.09 131.67,63.8 v124.77,63.8 | U4.32 v122.22,61.27
  Bottom 0.152: U3.15 82.5,44.4 82.3,44.4 78.74,40.84 72.44,40.84 68.89,44.4 59.74,44.4 U2.15 58.62,43.38 51,43.38 42.37,52.02 36.88,52.02 U1.12 | v87.88,49.89 90.32,52.32 92.56,52.32 96.32,56.08 98.86,56.08 101.19,58.42 106.27,58.42 107.49,59.64 120.6,59.64 U4.32 | v149.05,69.09 153.62,73.66 U5.3 | v122.22,61.27 v124.77,63.8
D3  (via drill 0.35)
  Top 0.152: SV3.4 177.8,71.42 169.37,79.86 162.46,79.86 v155.55,72.95 | v46.13,53.34 37.29,62.18 36.88,62.18 U1.8 | v149.05,68.07 136.55,68.07 v129.64,61.16
  Bottom 0.152: v155.55,72.95 153.72,71.12 U5.4 152.09,71.12 v149.05,68.07 | 100.23,54.3 100.28,54.25 100.28,44.2 98.04,41.96 97.84,41.96 U3.17 | 100.23,54.3 98.86,55.68 96.72,55.68 91.95,50.9 90.53,50.9 85.14,45.52 81.48,45.52 77.93,41.96 74.98,41.96 U2.17 68.38,48.46 51,48.46 v46.13,53.34 | 100.23,54.3 101.6,55.68 106.07,55.68 109.22,58.83 114.91,58.83 116.53,57.2 120.6,57.2 U4.31 120.7,57.2 121.01,57.2 124.97,61.16 v129.64,61.16
D4  (via drill 0.35)
  Top 0.152: v132.49,61.57 146.61,61.57 153.62,68.58 U5.5 | SV3.5 177.8,68.89 169.37,77.32 v162.46,77.32 | v90.83,51.61 90.83,51.41 U3.18 97.84,44.5 98.86,44.5 102.41,48.06 v102.41,48.77 | v72.44,43.38 73.66,43.38 74.68,44.4 74.88,44.4 U2.18 | v106.58,50.8 v115.21,50.8
  Bottom 0.152: v132.49,61.57 125.58,54.66 120.7,54.66 U4.30 120.6,54.56 118.97,54.56 v115.21,50.8 | v162.46,77.32 153.72,68.58 U5.5 | v90.83,51.61 90.63,51.61 84.94,45.92 81.28,45.92 79.86,44.5 74.98,44.5 U2.18 | v72.44,43.38 67.77,48.06 49.38,48.06 44.2,53.24 44.2,57 36.88,64.31 36.88,64.72 U1.7 | v106.58,50.8 104.44,50.8 v102.41,48.77
D5  (via drill 0.35)
  Top 0.152: v151.79,65.63 151.99,65.43 151.99,60.86 150.27,59.13 142.85,59.13 135.84,52.12 120.7,52.12 U4.29 v115.82,56.9 | SV3.6 175.56,66.04 169.06,72.54 163.07,72.54 162.66,72.95 v157.07,72.95 | v80.47,46.94 81.48,45.92 v87.17,45.92 | v68.68,39.73 70.92,41.96 70.92,42.98 U2.19 | v101.4,48.06 98.86,48.06 U3.19
  Bottom 0.152: U5.6 153.62,66.04 153.21,65.63 v151.79,65.63 151.59,65.84 151.59,69.39 151.99,69.8 153.92,69.8 v157.07,72.95 | v80.47,46.94 74.98,46.94 U2.19 | v87.17,45.92 96.72,45.92 U3.19 | v68.68,39.73 67.46,38.51 65.43,38.51 62.69,35.76 51,35.76 50.39,36.37 50.39,38.1 40.23,48.26 35.97,48.26 35.15,49.07 35.15,57.61 36.78,59.23 36.78,59.64 U1.9 | v115.82,56.9 114.3,58.42 113.69,58.42 107.29,52.02 107.29,49.28 106.07,48.06 v101.4,48.06
D6  (via drill 0.35)
  Top 0.152: v151.28,61.16 150.67,60.55 v132.49,60.55 130.05,60.55 129.95,60.45 127.1,60.45 121.72,65.84 104.34,65.84 101.7,63.2 v101.7,57.71 | v174.14,59.84 157.38,59.84 153.72,63.5 U5.7 | v77.62,52.43 74.98,49.78 74.98,49.58 U2.20 76.61,47.85 76.61,43.99 76,43.38 74.27,43.38 73.56,42.67 v71.63,42.67 | 94.18,53.14 v92.35,53.14 | U3.20 94.18,53.14 | v99.77,55.78 96.83,55.78 94.18,53.14
  Bottom 0.152: v132.49,60.55 121.51,49.58 120.7,49.58 U4.28 | v151.28,61.16 153.62,63.5 U5.7 | v174.14,59.84 SV3.7 | v77.62,52.43 80.77,52.43 81.48,53.14 v92.35,53.14 | v71.63,42.67 68.78,45.52 51.31,45.52 39.73,57.1 36.88,57.1 U1.10 | v99.77,55.78 v101.7,57.71
D7  (via drill 0.35)
  Top 0.152: v68.68,40.74 70.51,42.57 70.51,47.65 U2.21 | v174.14,57.3 157.38,57.3 157.33,57.35 | 157.33,57.35 153.72,60.96 U5.8 | U3.21 97.84,52.12 98.75,52.12 101.4,54.76 102.01,54.76 103.23,53.54 113.59,53.54 120.09,47.04 120.6,47.04 U4.27 v122.53,45.11 | v150.77,41.05 151.49,41.76 153.82,41.76 157.28,45.21 157.28,57.3 157.33,57.35
  Bottom 0.152: U1.13 36.88,49.48 42.37,49.48 51.41,40.44 64.72,40.44 66.24,38.91 66.85,38.91 v68.68,40.74 68.68,40.64 70.21,40.64 71.83,39.01 80.16,39.01 80.87,39.73 80.87,42.37 81.89,43.38 83.62,43.38 90.73,50.49 96.22,50.49 U3.21 | v174.14,57.3 SV3.8 | v150.77,41.05 148.34,41.05 145.39,43.99 123.65,43.99 v122.53,45.11
GND  (via drill 0.35)
  Top 0.254: JP2.6 143.36,80.06 143.36,77.62 JP3.6 143.36,77.52 v139.5,73.66 | U5.38 168.96,73.66 168.96,76.2 U5.39 | U2.3 59.74,74.98 59.74,77.42 U2.2 59.74,77.52 59.74,79.96 U2.1 | U3.1 82.6,79.96 82.6,77.52 U3.2 82.7,77.52 97.74,77.52 U3.31 97.84,77.42 97.84,74.98 U3.30 | RN2.1 127,49.99 122.33,49.99 121.31,51 119.48,51 105.77,64.72 105.46,64.72 U4.7 | v139.5,67.36 137.36,67.36 133.4,63.4 QG2.4 | IC6.7 97.13,12.7 93.98,9.55 U6.16 | IC6.13 105.46,25.4 105.46,22.86 IC6.12 105.36,22.76 105.36,22.45 103.63,20.73 103.63,19.61 105.36,17.88 IC6.10 105.46,17.78 105.46,15.24 IC6.9 105.56,15.24 108.1,12.7 IC7.7 113.08,12.6 114.1,11.58 121.72,11.58 122.43,12.29 122.43,13.61 126.29,17.48 S3.1 | 10.87,79.25 15.75,79.25 LED2.C | 10.87,79.25 10.16,79.96 JP22.1 10.26,80.06 10.26,81.58 11.38,82.7 19.3,82.7 24.89,77.11 24.89,73.36 23.57,72.03 S1.3 | 10.87,79.25 10.87,79.15 10.26,78.54 10.26,77.52 JP18.1 JP23.1 10.06,74.88 10.06,72.24 10.36,71.93 10.36,67.77 C12.- 10.46,67.67 11.68,67.67 14.83,64.52 C10.2 15.14,64.41 15.14,49.28 | J1.2 14.43,5.18 14.43,11.28 J1.3 14.33,11.38 14.33,27.33 5.38,36.27 5.38,39.83 C11.- 5.38,39.93 5.38,45.92 6.3,46.84 U8.1 6.4,47.04 6.4,47.35 8.33,49.28 15.14,49.28 | 15.14,49.28 15.65,49.28 16.87,48.06 16.87,46.23 15.54,44.91 15.54,44.4 C9.2 | 21.03,37.29 21.84,37.29 22.86,36.27 C3.- 22.96,36.17 22.96,35.15 27.74,30.38 27.74,30.18 C1.2 | 21.03,37.29 20.42,37.29 19.71,36.58 19.71,35.76 21.13,34.34 21.13,29.97 C2.2 | 21.03,37.29 21.03,50.8 22.05,51.82 QG1.4 | 54.61,47.4 53.85,48.16 53.85,50.29 U1.29 | 54.61,47.4 59.64,42.37 59.64,41.96 U2.16 64.41,37.19 v64.41,35.87
  Top 0.254: IC2.11 44.5,20.32 44.5,22.86 IC2.12 44.5,22.96 44.5,23.16 46.23,24.89 46.23,33.12 51,37.9 52.73,37.9 53.85,39.01 53.85,42.27 53.14,42.98 51.41,42.98 50.29,44.09 50.29,44.81 51,45.52 52.73,45.52 54.61,47.4 | 52.22,11.58 52.22,10.97 55.88,7.32 U6.1 | 52.22,11.58 52.22,12.8 IC3.7 | IC2.7 42.27,12.7 43.38,11.58 52.22,11.58 | IC5.7 82.3,12.8 80.67,12.8 78.64,10.77 69.29,10.77 67.36,12.7 IC4.8
  Bottom 0.254: JP2.6 143.46,80.06 165,80.06 168.86,76.2 U5.39 | U2.30 74.88,74.98 59.74,74.98 U2.3 | RN2.1 127,53.95 133.3,60.25 133.3,63.3 QG2.4 | U3.30 101.4,71.32 106.07,71.32 107.19,70.21 107.19,66.95 105.46,65.23 105.46,64.82 U4.7 | U3.1 81.48,81.08 73.86,81.08 72.85,80.06 59.74,80.06 U2.1 59.64,80.06 54.15,80.06 51.82,82.4 32.72,82.4 23.57,73.25 23.57,72.14 S1.3 23.47,72.03 23.47,64.72 23.16,64.41 C4.- 23.06,64.31 22.05,63.3 22.05,51.82 QG1.4 | v139.5,67.36 v139.5,73.66 | SV4.12 177.8,20.73 170.08,28.45 170.08,31.9 168.96,33.02 U5.22 | U5.25 168.96,40.64 168.96,39.73 170.08,38.61 170.08,34.24 168.96,33.12 U5.22 | U5.22 168.86,32.92 153.82,32.92 U5.19 153.72,33.02 153.72,30.58 U5.20 153.72,30.48 148.64,25.4 IC8.10 148.54,25.3 148.54,25.09 143.56,20.12 141.53,20.12 S2.1 141.43,20.02 139.7,20.02 136.55,16.87 124.46,16.87 121.41,13.82 116.33,13.82 115.32,12.8 113.08,12.8 IC7.7 112.98,12.7 111.86,11.58 104.34,11.58 103.23,12.7 IC6.7 | IC5.7 82.3,12.8 87.07,12.8 90.73,9.14 92.15,9.14 93.98,7.32 U6.16 | IC8.1 125.78,25.4 125.78,20.62 126.29,20.12 S3.1 | v64.41,35.87 65.84,34.44 76.3,34.44 82.5,40.64 82.5,41.86 U3.16 | VR2.1 41.76,3.35 36.88,8.23 36.88,12.7 IC2.7 36.78,12.8 31.6,17.98 28.65,17.98 | 28.65,17.98 25.5,17.98 24.89,17.37 24.89,16.56 22.25,13.92 22.25,11.48 IC1.1 | IC4.8 61.87,12.7 60.96,11.79 53.24,11.79 IC3.7 52.12,12.9 51.82,12.9 46.23,18.49 46.23,18.59 44.5,20.32 IC2.11 | 28.65,17.98 28.65,34.14 28.04,34.75 25.91,34.75 24.49,36.17 22.86,36.17 C3.-
LED0
  Top 0.152: DZ1.8 143.56,38.1 143.56,35.46 146,33.02 IC8.12
LED1
  Top 0.152: DZ1.7 141.02,38.1 141.02,35.46 143.46,33.02 IC8.13
LED2
  Top 0.152: DZ1.6 138.48,38.1 138.48,35.46 140.92,33.02 IC8.14
LED3
  Top 0.152: DZ1.5 135.94,38.1 135.94,35.46 138.38,33.02 IC8.15
LED4
  Top 0.152: DZ1.4 133.4,38.1 133.4,35.46 135.84,33.02 IC8.16
LED5
  Top 0.152: DZ1.3 130.86,38.1 130.86,35.46 133.3,33.02 IC8.17
LED6
  Top 0.152: DZ1.2 128.32,38.1 128.32,35.46 130.76,33.02 IC8.18
LED7
  Bottom 0.152: DZ1.1 125.78,38.1 125.78,36.17 128.22,33.73 128.22,33.02 IC8.19
N$1
  Top 0.152: R7.1 32.11,68.28 32.11,63.5 LED1.A
N$2
  Top 0.152: 24.89,26.31 27.74,26.31 R1.1 | 24.89,26.31 24.18,26.31 R2.2 24.89,26.31 | 24.89,26.31 24.89,13.82 29.77,8.94 IC1.7
N$3
  Top 0.152: C3.+ 20.83,35.36 26.62,29.57 26.62,29.06 28.14,27.53 28.75,27.53 28.96,27.33 28.96,20.02 25.91,16.97 VR1.2 | IC1.6 29.77,6.4 24.69,6.4 22.25,8.84 IC1.2
  Bottom 0.152: VR1.2 25.91,12.6 22.25,8.94 IC1.2
N$4
  Top 0.152: C1.1 30.68,30.07 30.68,28.45 31.8,27.33 31.8,5.79 29.87,3.86 IC1.5
N$5
  Top 0.152: SW3.1 6.3,20.83 6.3,23.98 4.37,25.91 4.37,31.6 D3.A
N$6
  Top 0.152: R2.1 21.34,26.21 21.34,19 23.37,16.97 VR1.1
N$8
  Top 0.152: J1.1_1 3.45,5.18 3.45,11.28 J1.1_2 3.45,11.38 3.45,14.22 8.84,19.61 8.84,20.73 SW3.2
N$9
  Top 0.152: LED2.A 15.75,71.22 15.44,70.92 R3.1
N$10  (via drill 0.35)
  Top 0.152: v100.58,17.37 100.58,15.95 98.86,14.22 96.62,14.22 92.66,10.26 69.09,10.26 68.99,10.36 60.15,10.36 58.12,12.39 58.12,15.75 59.74,17.37 59.74,17.88 IC3.10 | v108.31,20.73 112.98,25.4 IC7.2 113.08,25.4 113.08,27.94 IC7.1
  Bottom 0.152: v100.58,17.37 100.99,17.37 102.92,19.3 106.88,19.3 v108.31,20.73
N$11
  Top 0.152: DZ1.20 125.78,45.72 125.78,46.13 129.54,49.89 RN2.2
N$12
  Top 0.152: IC7.5 113.08,17.78 113.08,20.32 IC7.4
  Bottom 0.152: IC3.12 59.84,22.96 65.13,22.96 66.65,21.44 111.86,21.44 112.98,20.32 IC7.4
N$13
  Top 0.152: DZ1.19 128.32,45.72 128.32,46.13 132.08,49.89 RN2.3
N$14
  Top 0.152: 120.7,22.86 122.33,21.23 122.33,14.83 120.7,13.21 120.7,12.7 IC7.8 | 120.7,22.86 120.7,25.4 IC7.13 | 120.7,22.86 IC7.12
N$15
  Top 0.152: DZ1.18 130.86,45.72 130.86,46.13 134.62,49.89 RN2.4
N$16
  Top 0.152: R9.1 161.75,19.51 157.99,19.51 LED3.C | R9.1
N$17
  Top 0.152: R9.2 162.05,16.46 159.61,16.46 157.68,18.39 129.74,18.39 125.58,22.55 124.56,22.55 122.33,24.79 122.33,25.81 121.72,26.42 119.58,26.42 118.97,25.81 118.97,21.95 120.6,20.32 IC7.11
N$18
  Top 0.152: DZ1.17 133.4,45.72 133.4,46.13 137.16,49.89 RN2.5
N$19  (via drill 0.35)
  Top 0.152: R5.1 128.73,12.7 130.25,14.22 140.31,14.22 141.53,15.44 S2.3 | v87.07,3.96 72.03,3.96 70,5.99 70,8.13 68.58,9.55 59.74,9.55 56.69,12.6 56.69,16.87 59.74,19.91 59.74,20.42 IC3.11
  Bottom 0.152: v87.07,3.96 130.05,3.96 141.53,15.44 S2.3
N$20  (via drill 0.35)
  Top 0.152: R8.2 145.59,12.7 144.27,11.38 129.74,11.38 v129.54,11.58 | v57.4,18.59 57.4,22.66 59.74,24.99 59.74,25.5 IC3.13 | v57.4,16.05 57.4,12.5 59.94,9.96 68.78,9.96 69.29,9.45 v81.38,9.45
  Bottom 0.152: v129.54,11.58 129.54,12.19 126.29,15.44 S3.3 126.29,15.34 116.33,5.38 83.31,5.38 82.7,5.99 82.7,8.13 v81.38,9.45 | v57.4,16.05 v57.4,18.59
N$22
  Top 0.152: DZ1.16 135.94,45.72 135.94,46.13 139.7,49.89 RN2.6
N$23
  Top 0.152: DZ1.15 138.48,45.72 138.48,46.13 142.24,49.89 RN2.7
N$24
  Top 0.152: DZ1.14 141.02,45.72 141.02,46.13 144.78,49.89 RN2.8
N$25
  Top 0.152: DZ1.13 143.56,45.72 143.56,46.13 147.32,49.89 RN2.9
PA0  (via drill 0.35)
  Top 0.152: v24.89,39.52 24.89,35.87 26.01,34.75 28.14,34.75 32.41,30.48 32.41,19.3 34.75,16.97 34.75,12.7 37.59,9.86 50.9,9.86 v56.29,4.47
  Bottom 0.152: v24.89,39.52 25.3,39.93 25.3,73.66 33.12,81.48 39.93,81.48 42.88,78.54 106.48,78.54 107.09,77.93 107.09,77.01 106.48,76.4 104.75,76.4 103.73,75.39 103.73,74.47 105.36,72.85 105.36,72.44 U4.4 | v56.29,4.47 68.38,4.47 71.12,7.21 U6.7
PA1  (via drill 0.35)
  Top 0.152: v145.49,55.68 145.49,53.85 150.06,49.28 150.06,37.59 153.52,34.14 154.13,34.14 154.84,33.43 154.84,32.61 154.13,31.9 151.79,31.9 148.95,34.75 148.23,34.75 147.52,34.04 147.52,28.55 151.59,24.49 v151.59,23.06 | v76.2,4.67 73.66,7.21 U6.8
  Bottom 0.152: v145.49,55.68 145.49,57.71 145.09,58.12 144.78,58.12 131.98,70.92 119.99,70.92 116.03,74.88 105.46,74.88 U4.3 | v151.59,23.06 151.59,21.74 133.1,3.25 77.62,3.25 v76.2,4.67
PA2  (via drill 0.35)
  Top 0.152: v54.46,7.32 v51.21,10.57
  Bottom 0.152: v51.21,10.57 45.52,16.26 43.89,16.26 42.77,17.37 42.77,19 37.9,23.88 36.27,23.88 33.93,26.21 33.93,41.45 28.35,47.04 28.35,64.01 31.39,67.06 31.39,76.71 35.76,81.08 39.73,81.08 44.4,76.4 98.86,76.4 99.87,77.42 105.36,77.42 U4.2 | v54.46,7.32 54.46,5.28 55.98,3.76 72.75,3.76 76.2,7.21 U6.9
PA3  (via drill 0.35)
  Top 0.152: v157.99,45.52 157.99,44.6 155.25,41.86 v155.25,29.97
  Bottom 0.152: v157.99,45.52 154.13,49.38 153.52,49.38 146.61,56.29 146.61,68.28 138.89,76 119.99,76 116.03,79.96 105.46,79.96 U4.1 | v155.25,29.97 142.14,16.87 137.26,16.87 125.37,4.98 80.97,4.98 78.74,7.21 U6.10
PA4  (via drill 0.35)
  Top 0.152: v114.81,74.17 U4.40 | v114.81,61.47 114.81,58.52 v114,57.71 | v101.4,28.04 101.4,27.53 100.28,26.42 100.28,19.3 102.01,17.58 102.01,14.83 100.89,13.72 96.72,13.72 92.56,9.55 83.52,9.55 81.28,7.32 U6.11
  Bottom 0.152: v114.81,61.47 v114.81,74.17 | v114,57.71 114,56.79 107.7,50.49 107.7,42.06 106.07,40.44 104.34,40.44 101.4,37.49 v101.4,28.04
PA5  (via drill 0.35)
  Top 0.152: v116.53,73.36 U4.39 | v116.53,61.47 116.53,58.73 v114.71,56.9 | v117.14,39.73 117.14,37.59 105.97,26.42 104.34,26.42 103.12,25.2 103.12,18.09 v103.23,17.98 | v94.28,13.51 92.76,13.51 90.83,11.58 v85.55,11.58
  Bottom 0.152: v116.53,61.47 v116.53,73.36 | v114.71,56.9 113.39,55.58 113.39,43.48 v117.14,39.73 | v103.23,17.98 102.82,17.98 101.09,16.26 95.91,16.26 94.28,14.63 v94.28,13.51 | v85.55,11.58 85.55,9.04 83.82,7.32 U6.12
PA6  (via drill 0.35)
  Top 0.152: v34.04,16.66 34.04,12.8 39.73,7.11 v45.01,7.11
  Bottom 0.152: v34.04,16.66 29.26,21.44 29.26,35.97 27.94,37.29 26.01,37.29 24.18,39.12 24.18,39.83 24.89,40.54 24.89,73.86 32.92,81.89 40.13,81.89 43.08,78.94 112.57,78.94 116.53,74.98 120.6,74.98 U4.38 | v45.01,7.11 48.77,3.35 73.86,3.35 75.89,5.38 76.71,5.38 77.62,6.3 77.62,8.43 79.55,10.36 83.31,10.36 85.24,12.29 85.85,12.29 86.36,11.79 U6.13
PA7  (via drill 0.35)
  Top 0.152: v157.68,31.39 v157.68,43.28 | v133.2,5.38 93.47,5.38 92.56,6.3 92.56,8.43 91.85,9.14 90.73,9.14 88.9,7.32 U6.14
  Bottom 0.152: v157.68,43.28 154.13,46.84 153.52,46.84 152.5,47.85 152.5,48.26 146.2,54.56 146.2,59.64 133.5,72.34 120.7,72.34 U4.37 | v157.68,31.39 147.62,21.34 147.52,21.34 142.85,16.66 142.85,15.04 v133.2,5.38
PB0
  Bottom 0.152: IC8.9 145.59,25.4 139.7,31.29 127.91,31.29 126.8,32.41 126.8,34.54 123.04,38.3 107.09,38.3 105.66,36.88 105.46,36.88 U4.18
PB1
  Bottom 0.152: IC8.8 143.05,25.4 141.33,23.67 127.91,23.67 126.8,24.79 126.8,26.42 122.53,30.68 112.98,30.68 109.42,34.24 105.46,34.24 U4.19
PB2
  Bottom 0.152: U4.20 105.36,31.8 105.36,32.21 103.73,33.83 103.73,34.75 104.75,35.76 117.45,35.76 119.58,37.9 122.83,37.9 124.66,36.07 124.66,32 127,29.67 136.65,29.67 140.92,25.4 IC8.7
PB3
  Top 0.152: IC8.6 137.97,25.4 136.25,27.13 127.1,27.13 122.53,31.7 120.7,31.7 U4.21
PB4
  Top 0.152: U4.22 120.7,34.24 122.43,34.24 129.13,27.53 138.38,27.53 139.5,26.42 139.5,24.38 138.79,23.67 137.67,23.67 135.94,25.4 IC8.5
PB5
  Bottom 0.152: IC8.4 132.89,25.4 129.03,29.26 126.8,29.26 123.75,32.31 123.75,36.37 123.34,36.78 120.7,36.78 U4.23
PB6  (via drill 0.35)
  Top 0.152: v123.04,36.07 123.04,36.98 U4.24
  Bottom 0.152: IC8.3 130.35,25.4 126.9,28.85 126.59,28.85 123.04,32.41 v123.04,36.07
PB7
  Top 0.152: U4.25 120.6,41.86 120.6,41.45 118.97,39.83 118.97,31.29 121.31,28.96 124.66,28.96 128.22,25.4 IC8.2
PC5  (via drill 0.35)
  Top 0.152: v92.35,20.12 93.67,21.44 93.67,29.87 103.53,39.73 103.53,49.78 105.36,51.61 105.36,52.02 U4.12 | v80.16,17.88 80.16,13.01 78.44,11.28 69.9,11.28 v69.39,11.79
  Bottom 0.152: v92.35,20.12 91.75,20.12 90.53,18.9 81.18,18.9 v80.16,17.88 | v69.39,11.79 68.48,11.79 65.84,9.14 65.33,9.14 63.5,7.32 U6.4
PC6  (via drill 0.35)
  Top 0.152: v98.15,30.48 94.08,26.42 94.08,19.91 90.53,16.36 86.26,16.36 v84.73,14.83
  Bottom 0.152: v98.15,30.48 98.25,30.58 98.25,32.11 100.69,34.54 100.69,49.48 105.36,54.15 105.36,54.56 U4.11 | v84.73,14.83 83.92,14.83 83.11,14.02 72.75,14.02 66.04,7.32 U6.5
PC7  (via drill 0.35)
  Top 0.152: v98.96,53.34 102.72,57.1 105.36,57.1 U4.10 | v64.62,31.6 64.62,18.39 66.75,16.26 68.38,16.26 71.73,12.9 v71.73,11.99
  Bottom 0.152: v98.96,53.34 98.96,53.03 99.47,52.53 99.47,46.53 98.45,45.52 88.29,45.52 76.2,33.43 66.45,33.43 v64.62,31.6 | v71.73,11.99 71.73,10.46 68.58,7.32 U6.6
RCLK
  Top 0.152: U5.15 153.62,43.18 153.62,44.2 152.5,45.31 152.5,57.3 153.62,58.42 U5.9
RESET  (via drill 0.35)
  Top 0.152: IC3.3 52.22,23.06 52.22,25.5 IC3.2 | v152.3,69.09 150.88,70.51 137.16,70.51 134.01,67.36 120.7,67.36 U4.35 | v167.03,67.46 167.44,67.46 168.86,66.04 U5.35 168.96,66.04 174.96,60.05 v174.96,54.05 | v56.29,20.22 56.29,12.39 59.54,9.14 63.91,9.14 64.92,8.13 64.92,5.99 68.28,2.64 v161.85,2.64
  Bottom 0.152: v152.3,69.09 152.3,68.38 153.21,67.46 v167.03,67.46 | v174.96,54.05 176.68,52.32 178.41,52.32 179.53,51.21 179.53,32.61 177.8,30.89 SV4.8 179.53,28.75 179.53,19.91 162.25,2.64 v161.85,2.64 | v56.29,20.22 53.54,22.96 52.22,22.96 IC3.3
RX
  Top 0.152: JP2.2 133.2,80.06 133.2,77.62 JP3.2 138.99,71.83 150.16,71.83 151.99,70 153.82,70 154.84,68.99 154.84,68.17 154.13,67.46 153.52,67.46 152.5,66.45 152.5,60.55 153.21,59.84 153.82,59.84 154.84,58.83 154.84,58.01 153.72,56.9 153.72,55.88 U5.10
TX
  Top 0.152: JP3.3 135.74,77.62 135.74,80.06 JP2.3
  Bottom 0.152: U5.11 153.42,53.34 147.01,59.74 147.01,68.48 138.99,76.5 136.85,76.5 JP3.3

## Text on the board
tPlace: I/O XP | 2K | 10K | SST39SF040 | AS6C4008 | Z84C00xx | 4.7K | !NMI! | !INT! | !HALT! | 2.2K | 4.7K | 4.7K | 555 | 10K | 7.35" x 3.3"
tNames: RESET | A11 | A10 | *5V | *5V | PA3 | PA4 | D0 | *5V | 5V | GND | PA2 | PA5 | CPU | ROM | RAM | PPI | DTR / / RX / / TX / / 5V / / RTS / / GND | A14 | UART | PA1 | PA6 | A12 | A14 | A12 | !RAM_WE! | PA0 | PA7 | A15 | A7 | A13 | A7 | A13 | !IORD! | !IOWR! | CLK | A8 | A8 | !PPI! | RESET | RESET | D4 | A9 | A9 | *GND | D0 | D3 | A11 | A11 | A1 | D1 | 82C55 | 1.8432MHz | D7 | D5 | !ROM_OE! | !RAM_OE! | A0 | D2 | RCLK | D6 | A10 | A10 | PC7(E) | D3 | CLOCKS | 16C550 | RX | *5V | A0 | !ROM_CE! | !RAM_CE! | PC6(R/!W!) | D4 | TX | D2 | *GND | A0 | D7 | A0 | D7 | PC5(RS) | D5 | D7 | D0 | D0 | PC4 | D6 | 1MHz | A0 | D0 | PC0 | D7 | !M1! | !ENABLE_UART! | A1 | D1 | !RESET! | D2 | D2 | PC1 | *5V | RCLK | A2 | !BUSRQ! | *GND | *GND | PC2 | PB7 | !INT! | D3 | D3 | 1.8432MHz | !NMI! | !WAIT! | PC3 | PB6 | FAST | !HALT! | PB0 | PB5 | 7 6 5 4 3 2 1 0 | !WR! | SLOW | !MREQ! | !WR! | PB1 | PB4 | 1uF | !IORQ! | !RD! | PB2 | PB3 | *GND | !RD! | 74574 | 7414 | 74138 | 7432 | 7432 | 7400 | 7474 | D0 / / D1 / / D2 / / D3 / / D4 / / D5 / / D6 / / D7 / / A0 / / A1 / / A2 / / A3 / / A4 / / A5 / / A6 / / A7 / / !IORD! / / !IOWR! / / !IORQ! / / RESET / / !OTHER1! / / !OTHER2! / / 5V / / GND | INPUT: 7 TO 12V DC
